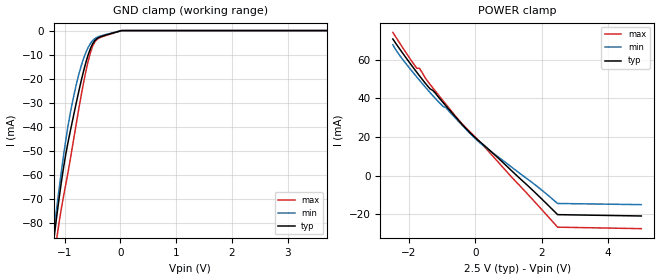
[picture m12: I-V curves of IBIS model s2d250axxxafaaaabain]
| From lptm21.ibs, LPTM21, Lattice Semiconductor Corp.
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|   Model s2d250axxxafaaaabain
[Model]   s2d250axxxafaaaabain
Model_type   Input
Polarity   Non-Inverting
Enable   Active-Low
Vinl =   1.0700V
Vinh =   1.4300V
C_comp   4.2000pF   3.8000pF   7.5000pF
[Temperature Range]   25.0000   0.1050k   -40.0000
[Voltage Range]   2.5000V   2.3800V   2.6300V
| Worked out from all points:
|   GND clamp passes 1 mA (typ) near -0.13 V on its own axis
[GND_clamp]
|Voltage   I(typ)   I(min)   I(max)
-2.5V     -558.7mA   -538.8mA   -577.3mA
-1.22V    -91.65mA   -88.51mA   -100.2mA
-1.18V    -84.01mA   -80.7mA    -92.85mA
-1.14V    -76.64mA   -73.08mA   -85.95mA
-1.02V    -56.82mA   -51.79mA   -68.7mA
-940mV    -46.33mA   -39.59mA   -58.84mA
-780mV    -28.68mA   -21.23mA   -36.93mA
-580mV    -10.13mA   -7.016mA   -12.79mA
-500mV    -5.522mA   -4.164mA   -6.524mA
-420mV    -3.293mA   -2.799mA   -3.655mA
20mV      0A         0A         0A
5V        0A         0A         0A
[POWER_clamp]
|Voltage   I(typ)   I(min)   I(max)
-2.48V    70.8mA     67.79mA    74.22mA
-2.24V    64.81mA    61.5mA     67.79mA
-1.76V    53.56mA    51.12mA    55.62mA
-1.68V    51.75mA    49.46mA    55.62mA
-1.36V    44.95mA    43.02mA    47.29mA
-1.2V     42.73mA    39.97mA    43.79mA
-960mV    37.69mA    35.72mA    38.61mA
-880mV    36.09mA    35.18mA    36.9mA
-480mV    28.21mA    27.66mA    28.47mA
0V        19.67mA    19.21mA    19.91mA
2.48V     -20.27mA   -14.48mA   -26.76mA
5V        -20.96mA   -15.08mA   -27.53mA
